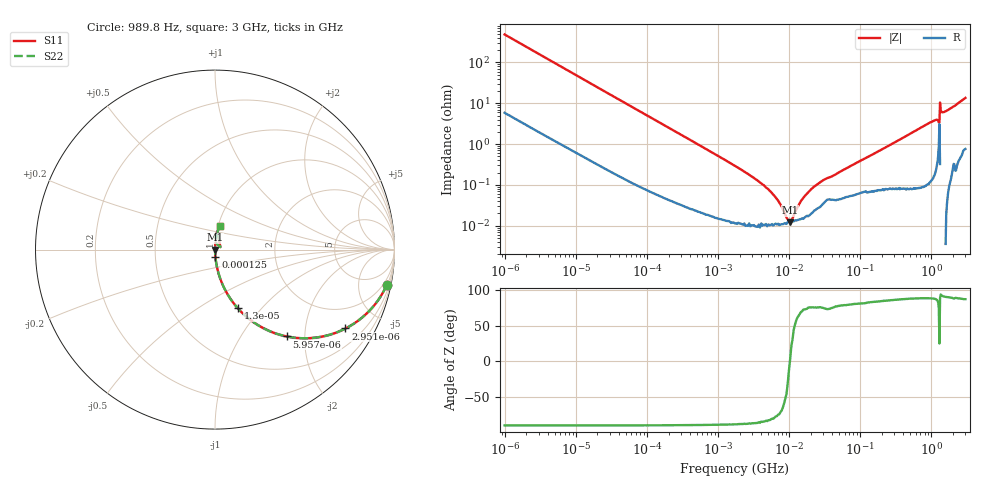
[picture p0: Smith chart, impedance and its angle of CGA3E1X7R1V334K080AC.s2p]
! S-Parameter Data Generated by TDK Corporation
! Copyright(C) 2020 TDK Corporation.
! All Rights Reserved.
! TDK P/N: CGA3E1X7R1V334K080AC (Multilayer Ceramic Chip Capacitor)
! Property: C=330nF
! Size(LxWxT): 1.6x0.8x0.8mm
! Model Type: s2p (Touchstone File Format Version 1.0)
! Frequency: DC=Yes Start=0.000989846MHz Stop=3000MHz 463points Log-sweep
! Model Generated on Aug. 18, 2020
! Port Assignments:
!  1 ---| |--- 2
! Applicable Conditions:
!  Temperature = 25 degC
!  DC Bias Voltage = 0 V
!  Small Signal Operation
! Terms and conditions regarding TDK Simulation Models
! (1)This simulation model is being provided solely for informational purposes. Please refer to the specifications of the products in terms of detailed characteristics of such products.
! (2)In no event shall TDK Corporation of any of its subsidiaries be liable for any loss or damage arising, directly or indirectly,
!  From any information contained in this simulation model, including, but not limited to loss or damages arising from any inaccuracies, omissions or errors in connection with such information.
! (3)Any and all copyrights on this simulation model are owned by TDK Corporation.
!  Duplication or redistribution of this simulation model without prior written permission from TDK Corporation is prohibited.
! (4)This simulation model is subject to any modification or change without any prior notice.
! (5)Neither TDK Corporation nor any of its subsidiaries shall make any warranty, express or implied,
!  Including but not limited to the correctness, implied warranties of merchantability and fitness for a particular purpose with respect to this simulation models.
! (6)The use of this simulation model shall be deemed to have consented to the terms and conditions hereof.
# Hz S MA R 50
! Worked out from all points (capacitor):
!   462 points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, 989.8 Hz to 3 GHz, reference 50 ohm
!   read as one part in series: C = 330 nF near 1.07 kHz
!   lowest |Z| = 12.2 mohm at 10.27 MHz (marker M1)
!   series resonance near 10.21 MHz, so ESL is about 740 pH
!   S11 on the Smith chart (normalised r, x): 989.8 Hz: 1.12, -9.72; 2.951 kHz: 1.04, -3.28; 5.957 kHz: 1.02, -1.63; 13 kHz: 1.01, -0.75; 125 kHz: 1.00, -0.08; 3 GHz: 1.02, +0.27
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989.846  0.9772 -11.6  0.201 77.7  0.201 77.7  0.9772 -11.6
2951.47  0.8495 -31.2  0.5174 58.1  0.5174 58.1  0.8495 -31.2
5957.379  0.6291 -50.3  0.7696 39.0  0.7696 39.0  0.6291 -50.3
12024.64  0.3757 -67.2  0.922 22.1  0.922 22.1  0.3757 -67.2
13000.58  0.3514 -68.7  0.9318 20.6  0.9318 20.6  0.3514 -68.7
35854.41  0.137 -81.4  0.9888 7.9  0.9888 7.9  0.137 -81.4
124966.8  0.04033 -86.8  0.9986 2.3  0.9986 2.3  0.04033 -86.8
146075.1  0.03457 -87.1  0.9989 2.0  0.9989 2.0  0.03457 -87.1
1774518  0.002842 -87.5  0.9999 0.2  0.9999 0.2  0.002842 -87.5
5291161  0.0007195 -81.9  0.9999 0.0  0.9999 0.0  0.0007195 -81.9
7229596  0.0003682 -73.6  0.9999 0.0  0.9999 0.0  0.0003682 -73.6
9500176  0.0001433 -30.9  0.9999 0.0  0.9999 0.0  0.0001433 -30.9
1.027123e7  0.000122 2.6  0.9999 -0.0  0.9999 -0.0  0.000122 2.6
1.517317e7  0.0004437 70.0  0.9998 -0.0  0.9998 -0.0  0.0004437 70.0
2.073191e7  0.0008102 75.5  0.9998 -0.0  0.9998 -0.0  0.0008102 75.5
3.062619e7  0.001334 74.3  0.9996 -0.1  0.9996 -0.1  0.001334 74.3
2.507343e8  0.009122 84.5  0.9992 -0.5  0.9992 -0.5  0.009122 84.5
1.017911e9  0.03563 85.8  0.998 -2.0  0.998 -2.0  0.03563 85.8
1.243477e9  0.03734 79.7  0.994 -2.1  0.994 -2.1  0.03734 79.7
1.374365e9  0.06248 88.8  1.001 -3.6  1.001 -3.6  0.06248 88.8
1.581072e9  0.06338 86.3  0.998 -3.6  0.998 -3.6  0.06338 86.3
3e9  0.1333 79.1  0.9836 -7.6  0.9836 -7.6  0.1333 79.1
